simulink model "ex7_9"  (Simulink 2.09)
settings: Solver=ode45  StartTime=0.0  StopTime=10.0  RelTol=1e-3  AbsTol=1e-6

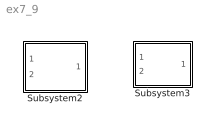
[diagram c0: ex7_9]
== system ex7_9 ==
  Subsystem2 : Subsystem
  Subsystem3 : Subsystem

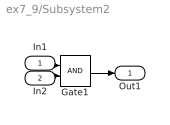
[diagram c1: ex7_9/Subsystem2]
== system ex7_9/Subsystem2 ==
  In1 : Inport  Port=1  PortWidth=-1  SampleTime=-1
  In2 : Inport  Port=2  PortWidth=-1  SampleTime=-1
  Gate1 : Logic  Operator=AND  Inputs=2
  Out1 : Outport  Port=1  InitialOutput=0
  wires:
  In1/1 -> Gate1/1
  Gate1/1 -> Out1/1
  In2/1 -> Gate1/2

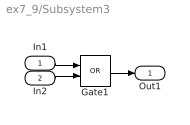
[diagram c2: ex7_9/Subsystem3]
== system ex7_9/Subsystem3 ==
  In1 : Inport  Port=1  PortWidth=-1  SampleTime=-1
  In2 : Inport  Port=2  PortWidth=-1  SampleTime=-1
  Gate1 : Logic  Operator=OR  Inputs=2
  Out1 : Outport  Port=1  InitialOutput=0
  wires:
  In1/1 -> Gate1/1
  Gate1/1 -> Out1/1
  In2/1 -> Gate1/2
